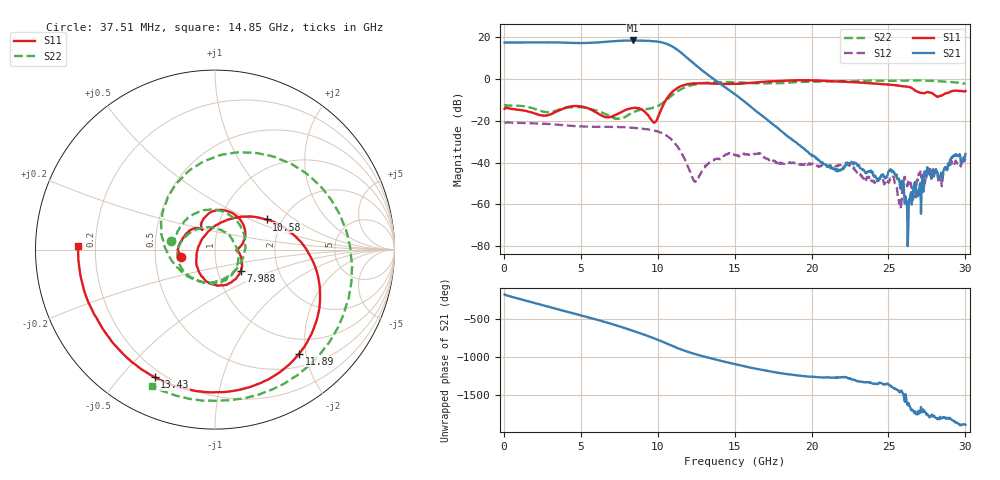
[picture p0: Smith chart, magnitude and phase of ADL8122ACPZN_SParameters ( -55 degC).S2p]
! "Analog Devices, Inc."
! Device:	ADL8122ACPZN
! Description:	"10 kHz to 10 GHz, Wideband, Low Noise Amplifier"
! Conditions:	Vdd = 5.0 V
!		IDQ = 95 mA
!		Pin = -25 dBm
!		Operating Temperature = +25 C (at package bottom)
! Product validation unit SN1 soldered down to Evaluation Board as shown on ADL8122-EVALZ User Guide. Board loss de-embedded from S21 magnitude.  All other RF measurements reference to RF coaxial connector.
! Frequency (GHz)	S11_Mag (dB)	S11_Phase (deg)	S21_Mag (dB)	S21_Phase (deg)	S12_Mag (dB)	S12_Phase (deg)	S22_Mag (dB)	S22_Phase (deg)
#  GHZ  S  DB  R 50
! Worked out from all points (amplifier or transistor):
!   800 points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, 37.51 MHz to 30 GHz, reference 50 ohm
!   highest |S21| = 18.5 dB at 8.363 GHz (marker M1)
!   |S21| within 3 dB of that: start of sweep to 10.97 GHz
!   unconditionally stable (mu >= 1): start of sweep to end of sweep
!   at 5.025 GHz: K = 1.15, MAG = 17.6 dB, |S12| = -22.7 dB
!   at 15.04 GHz: K = 9.23, MAG = 1.8 dB, |S12| = -36.3 dB
!   at 30 GHz: K = 736.97, MAG = -30.6 dB, |S12| = -38.2 dB
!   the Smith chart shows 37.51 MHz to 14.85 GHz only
!   S11 on the Smith chart (normalised r, x): 37.51 MHz: 0.68, -0.06; 7.988 GHz: 1.29, -0.32; 10.58 GHz: 1.66, +0.63; 11.89 GHz: 0.72, -1.88; 13.43 GHz: 0.17, -0.62; 14.85 GHz: 0.14, +0.01
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0.03750899  -14.26 -167.4  17.42 -177.4  -20.86 3.1  -12.00 168.8
1.575009  -15.58 135.2  17.51 93.9  -21.16 -74.8  -13.44 72.7
2.250008  -17.08 123.6  17.54 57.0  -21.31 -107.3  -14.93 22.3
3.075008  -16.79 122.0  17.57 11.6  -21.64 -148.1  -15.69 -55.4
3.900008  -14.02 102.4  17.43 -33.3  -22.13 171.7  -14.01 -121.1
5.062508  -13.21 51.3  17.23 -95.0  -22.71 114.8  -13.55 -175.3
5.812507  -15.27 19.0  17.43 -135.7  -22.88 76.9  -14.65 159.6
6.675007  -18.34 -0.4  17.86 174.9  -22.89 31.6  -17.08 119.8
7.275007  -17.14 -9.6  18.20 138.4  -22.93 -1.3  -19.04 67.3
7.987507  -14.62 -39.6  18.43 92.3  -23.18 -41.9  -17.74 -10.1
8.362506  -13.92 -61.2  18.48 67.2  -23.31 -63.7  -16.11 -43.2
9.262506  -16.51 -128.1  18.36 3.9  -24.05 -117.3  -14.31 -103.1
10.05001  -17.50 89.5  17.85 -57.2  -25.32 -171.6  -12.65 -155.0
10.57501  -9.55 30.2  16.86 -101.8  -27.18 147.8  -9.98 160.3
11.13751  -4.93 -9.8  14.70 -150.0  -31.08 102.0  -6.59 106.3
11.88751  -2.54 -50.9  10.30 153.0  -40.85 39.5  -3.67 42.2
13.425  -2.09 -115.4  1.09 63.9  -39.80 -177.0  -1.62 -49.7
14.85  -2.36 178.4  -6.40 -6.2  -35.70 104.5  -1.55 -114.8
15.0375  -2.33 169.1  -7.39 -15.2  -36.30 98.7  -1.59 -122.7
20.025  -0.60 17.9  -36.95 -178.6  -40.69 -54.1  -1.30 49.0
25.0125  -2.68 -113.6  -44.13 75.1  -49.67 137.8  -0.87 -102.8
30  -5.74 -93.2  -35.92 -89.8  -38.15 -94.8  -2.20 -160.9
